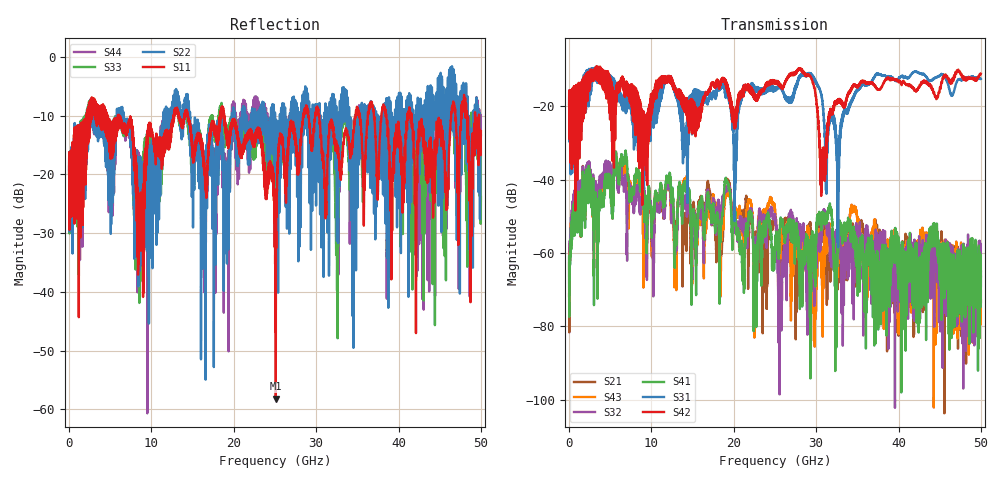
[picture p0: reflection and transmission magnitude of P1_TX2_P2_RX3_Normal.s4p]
!Keysight Technologies,N5225B,MY57041031,A.13.20.10
!Date: Friday, May 31, 2019 11:31:42
!Correction: S11(Full 4 Port(1,2,3,4))
!S12(Full 4 Port(1,2,3,4))
!S13(Full 4 Port(1,2,3,4))
!S14(Full 4 Port(1,2,3,4))
!S21(Full 4 Port(1,2,3,4))
!S22(Full 4 Port(1,2,3,4))
!S23(Full 4 Port(1,2,3,4))
!S24(Full 4 Port(1,2,3,4))
!S31(Full 4 Port(1,2,3,4))
!S32(Full 4 Port(1,2,3,4))
!S33(Full 4 Port(1,2,3,4))
!S34(Full 4 Port(1,2,3,4))
!S41(Full 4 Port(1,2,3,4))
!S42(Full 4 Port(1,2,3,4))
!S43(Full 4 Port(1,2,3,4))
!S44(Full 4 Port(1,2,3,4))
!S4P File: Measurements: <S11,S12,S13,S14>,
!<S21,S22,S23,S24>,
!<S31,S32,S33,S34>,
!<S41,S42,S43,S44>:
# Hz S  dB  R 50.0
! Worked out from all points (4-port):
!   5000 points, 10 MHz to 50 GHz, reference 50 ohm
!   strongest paths, dB at 10 MHz, 12.51 GHz, 25.01 GHz, 37.51 GHz, 50 GHz:
!     S42: -19.3, -14.3, -13.4, -15.4, -11.1
!     S31: -19.5, -13.0, -15.4, -11.1, -12.5
!     S41: -60.9, -43.5, -60.0, -66.8, -69.0
!     S32: -61.3, -46.4, -49.4, -62.5, -65.0
!     S43: -71.7, -46.2, -47.9, -57.9, -73.4
!     S21: -62.9, -45.1, -51.4, -55.7, -66.4
!   lowest |S11| = -58.2 dB at 25.1 GHz (marker M1), VSWR 1.00, Z = 50 + j0.119 ohm
!   |S11| at or under -10 dB: 6.091 GHz to 12.71 GHz (6.615 GHz wide, 70.4 % of centre); 18.82 GHz to 28.43 GHz (9.604 GHz wide, 40.7 % of centre); 41.58 GHz to 46.38 GHz (4.809 GHz wide, 10.9 % of centre)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
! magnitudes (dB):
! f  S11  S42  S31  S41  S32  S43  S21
! 10 MHz  -19.8  -19.3  -19.5  -60.9  -61.3  -71.7  -62.9
! 5.65 GHz  -10.5  -22.2  -14.4  -32.6  -32.4  -32.3  -32.4
! 25.1 GHz  -58.2  -13.1  -15.1  -57.3  -52.0  -51.9  -51.5
! 29.31 GHz  -14.3  -11.9  -11.0  -94.2  -63.9  -56.3  -55.4
! 30.78 GHz  -17.6  -33.5  -19.4  -50.0  -50.6  -64.6  -54.2
! 34.54 GHz  -12.6  -14.2  -17.3  -52.7  -64.0  -48.4  -52.9
! 50 GHz  -12.6  -11.1  -12.5  -69.0  -65.0  -73.4  -66.4
